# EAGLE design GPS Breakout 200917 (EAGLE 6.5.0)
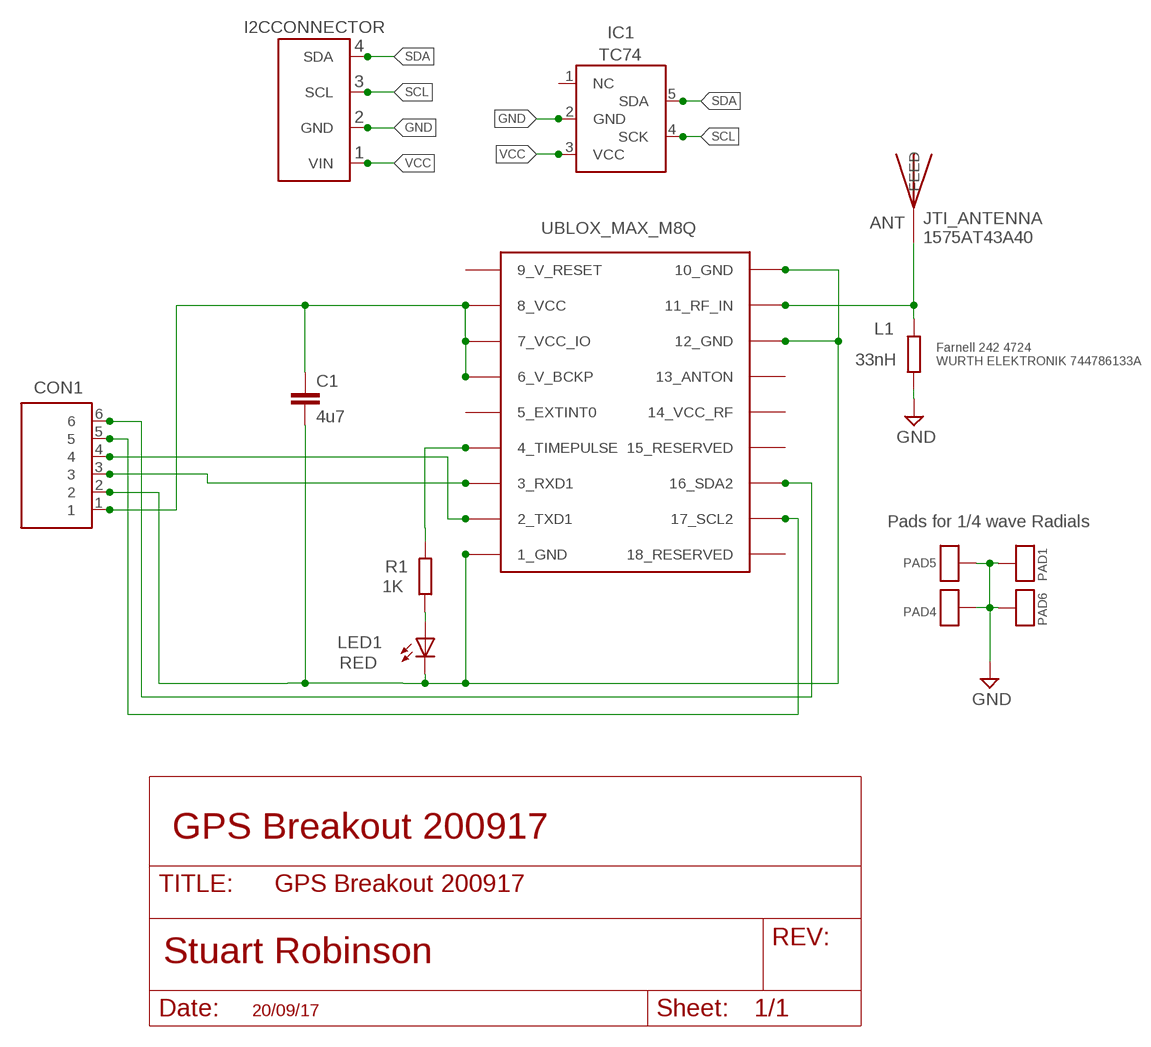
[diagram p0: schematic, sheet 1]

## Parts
ANT  JTI_ANTENNA-1575AT43A40  [JTI_ANTENNA-1575AT43A40]
C1  4u7  C-EUC0805  [C0805]
CON1  6X1  [6X1]
I2CCONNECTOR  BME280  [BME280]
IC1  TC74  [SOT23-5]
L1  33nH  R-EU_R0603  [R0603]
LED1  RED  0805LED  [0805LED]
PAD1  ANTPAD2  [ANTPAD2]
PAD4  ANTPAD2  [ANTPAD2]
PAD5  ANTPAD2  [ANTPAD2]
PAD6  ANTPAD2  [ANTPAD2]
R1  1K  R-EU_R0805  [R0805]
UBLOX_MAX_M8Q  UBLOX_MAX  [UBLOX_MAX]

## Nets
GND [GND]: C1.2 CON1.2 I2CCONNECTOR.GND IC1.2(GND) L1.1 LED1.C PAD1.P$1 PAD4.P$1 PAD5.P$1 PAD6.P$1 UBLOX_MAX_M8Q.1_GND UBLOX_MAX_M8Q.10_GND UBLOX_MAX_M8Q.12_GND
N$7: LED1.A R1.1
N$12: R1.2 UBLOX_MAX_M8Q.4_TIMEPULSE
RFIN: ANT.FEED L1.2 UBLOX_MAX_M8Q.11_RF_IN
RX: CON1.3 UBLOX_MAX_M8Q.3_RXD1
SCL: CON1.5 I2CCONNECTOR.SCL IC1.4(SCK) UBLOX_MAX_M8Q.17_SCL2
SDA: CON1.6 I2CCONNECTOR.SDA IC1.5(SDA) UBLOX_MAX_M8Q.16_SDA2
TX: CON1.4 UBLOX_MAX_M8Q.2_TXD1
VCC [gpspower]: C1.1 CON1.1 I2CCONNECTOR.VIN IC1.3(VCC) UBLOX_MAX_M8Q.6_V_BCKP UBLOX_MAX_M8Q.7_VCC_IO UBLOX_MAX_M8Q.8_VCC
Unconnected: IC1.1(NC) UBLOX_MAX_M8Q.5_EXTINT0 UBLOX_MAX_M8Q.13_ANTON UBLOX_MAX_M8Q.14_VCC_RF UBLOX_MAX_M8Q.15_RESERVED UBLOX_MAX_M8Q.18_RESERVED

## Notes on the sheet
- 4
- 3
- 2
- 1
- JTI_ANTENNA
  1575AT43A40
- Farnell 242 4724
  WURTH ELEKTRONIK 744786133A
- Pads for 1/4 wave Radials
- GPS Breakout 200917
- 20/09/17

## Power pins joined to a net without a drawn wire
9_V_RESET: UBLOX_MAX_M8Q.9_V_RESET

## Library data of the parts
ANT = Ava2:JTI_ANTENNA-1575AT43A40
C1 = resistor:C-EU: CAPACITOR, European symbol
CON1 = My_Pin_Headers:6X1
I2CCONNECTOR = LMA2:BME280
IC1 = LMA2:TC74
L1 R1 = resistor:R-EU_: RESISTOR, European symbol
LED1 = LMA2:0805LED
PAD1 PAD4-PAD6 = LMA2:ANTPAD2
UBLOX_MAX_M8Q = Ava2:UBLOX_MAX: UBLOX MAX

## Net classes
0 default: width 0.152 mm
1 GND: width 0.508 mm
2 gpsdefault: width 0.508 mm
3 gpspower: width 0.508 mm

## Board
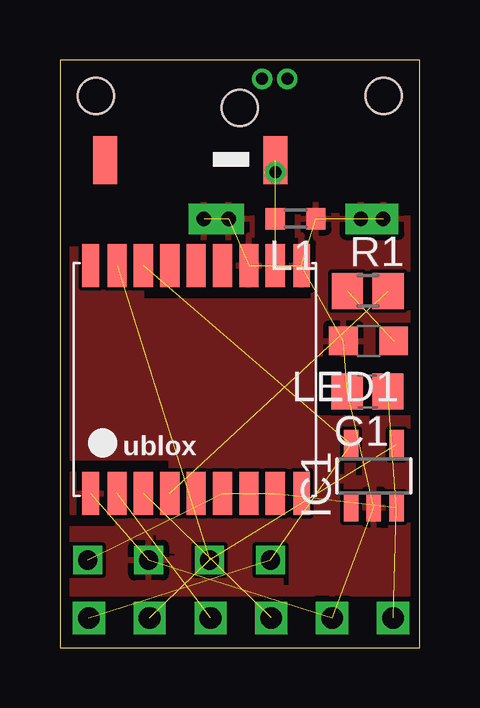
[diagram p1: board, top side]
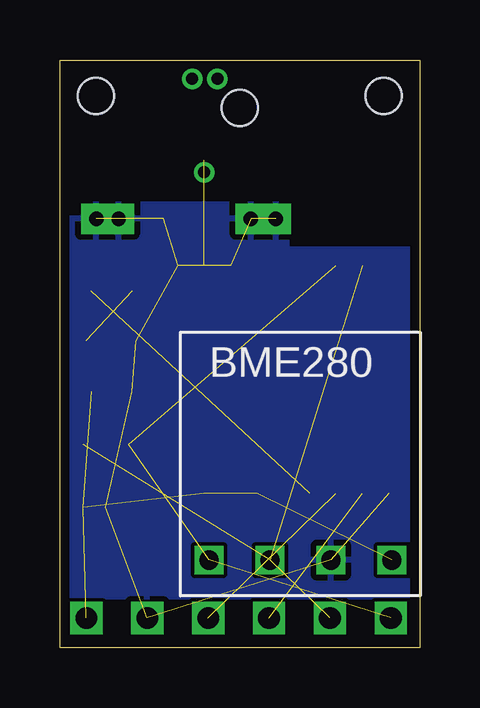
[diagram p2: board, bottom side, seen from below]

Size 15 x 24.5 mm. Coordinates in mm from the lower left corner, seen from the top.
Outline: 0,0 15,0 15,24.5 0,24.5 0,0
Copper layers (1*16): Top 0.0356mm / dielectric 1.5011mm / Bottom 0.0356mm
Design rules "LaenPCBOrder *": minimum track width 6mil, minimum drill 13mil, track to track 6mil, track to pad 6mil, pad to pad 6mil, via to via 6mil, smd to smd 6mil, copper to edge 15mil, drill to drill 6mil, minimum pad ring 7mil, minimum via ring 7mil, stop-mask expansion 4mil, vias tented up to drill 1000mil, thermal gap 10mil
Holes 1.5 mm at 1.5,23 7.5,22.5 13.5,23
tRestrict: area 0.4,16.8 to 5.4,18.5; area 8.4,18.4 to 8.5,18.6; area 8.4,16.9 to 8.6,17.4; area 9.3,16.9 to 9.5,17.4; area 9.5,18.4 to 9.5,18.6; area 11.3,18.1 to 11.7,18.6; area 7.9,18 to 8.4,18.7; area 9.5,18.1 to 10,18.6; area 12.4,17 to 13.7,17.3; area 14.4,18 to 14.6,18.6; area 3.5,14.6 to 10.4,15; area 0.5,7.3 to 4.5,7.8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
bRestrict: area 0.3,16.7 to 5.4,18.6; area 14.4,18 to 14.6,18.6

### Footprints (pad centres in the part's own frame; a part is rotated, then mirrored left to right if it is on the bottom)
JTI_ANTENNA-1575AT43A40 = smd 1 x 2: FEED -3.175,0; NC 3.925,0
C0805 = smd 1.3 x 1.5: 1 -0.85,0; 2 0.85,0
6X1 = drill 0.9 square: 1 -6.35,0; 2 -3.81,0; 3 -1.27,0; 4 1.27,0; 5 3.81,0; 6 6.35,0
BME280 = drill 0.8 square: GND -1.27,0; SCL 1.27,0; SDA 3.81,0; VIN -3.81,0
SOT23-5 = smd 0.6 x 1.2: 1 -0.95,-1.306; 2 0,-1.306; 3 0.95,-1.306; 4 0.95,1.306; 5 -0.95,1.306
R0603 = smd 0.8 x 0.9: 1 -0.85,0; 2 0.85,0
0805LED = smd 1.2 x 1.2: A 0,-1.05; C 0,1.05
ANTPAD2 = drill 0.6 pad 1.27 square: P$1 0,0
R0805 = smd 1.3 x 1.5: 1 -0.85,0; 2 0.85,0
UBLOX_MAX = smd 1.8 x 0.7: 1_GND 4.95,-4.45; 9_V_RESET 4.95,4.35; 10_GND -4.55,4.35; 18_RESERVED -4.55,-4.45 | smd 1.8 x 0.8: 2_TXD1 4.95,-3.35; 3_RXD1 4.95,-2.25; 4_TIMEPULSE 4.95,-1.15; 5_EXTINT0 4.95,-0.05; 6_V_BCKP 4.95,1.05; 7_VCC_IO 4.95,2.15; 8_VCC 4.95,3.25; 11_RF_IN -4.55,3.25; 12_GND -4.55,2.15; 13_ANTON -4.55,1.05; 14_VCC_RF -4.55,-0.05; 15_RESERVED -4.55,-1.15; 16_SDA2 -4.55,-2.25; 17_SCL2 -4.55,-3.35

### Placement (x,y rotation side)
ANT  5.81,20.32 180 top
C1  12.83,10.68 180 top
CON1  7.55,1.23 180 top
I2CCONNECTOR  4.97,3.65 180 bottom
IC1  13.09,7.16 0 top
L1  9.83,17.88 180 top
LED1  12.87,12.79 90 top
PAD1  12.55,17.88 0 top
PAD4  13.48,17.88 0 top
PAD5  7.04,17.88 0 top
PAD6  6,17.88 0 top
R1  12.84,14.87 0 top
UBLOX_MAX_M8Q  5.73,11.38 270 top

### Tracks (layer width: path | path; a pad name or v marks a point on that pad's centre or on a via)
GND  (12 unrouted)
  pour Top: 0.38,18.5 14.74,18.5 14.78,2.21 0.2,2.22 0.36,17.69
  pour Bottom: 0.5,18.5 14.68,18.5 14.79,2.11 0.5,2.11
N$1  (via drill 0.5)
  other vias: 8.43,23.71
N$3  (via drill 0.5)
  other vias: 8.98,19.82
N$6  (via drill 0.5)
  other vias: 9.48,23.71
N$7  (1 unrouted)
N$12  (1 unrouted)
RFIN  (2 unrouted)
RX  (1 unrouted)
SCL  (3 unrouted)
SDA  (3 unrouted)
TX  (1 unrouted)
VCC  (6 unrouted)

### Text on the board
Notes: ANT | L1 | R1 | LED1 | C | A | 200917 | C1 | UBLOX MAX M8Q | IC1 | VCC | GND | SCL | SDA | <I2C | 1 | SDA | SCL | TX | RX | GND | VCC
